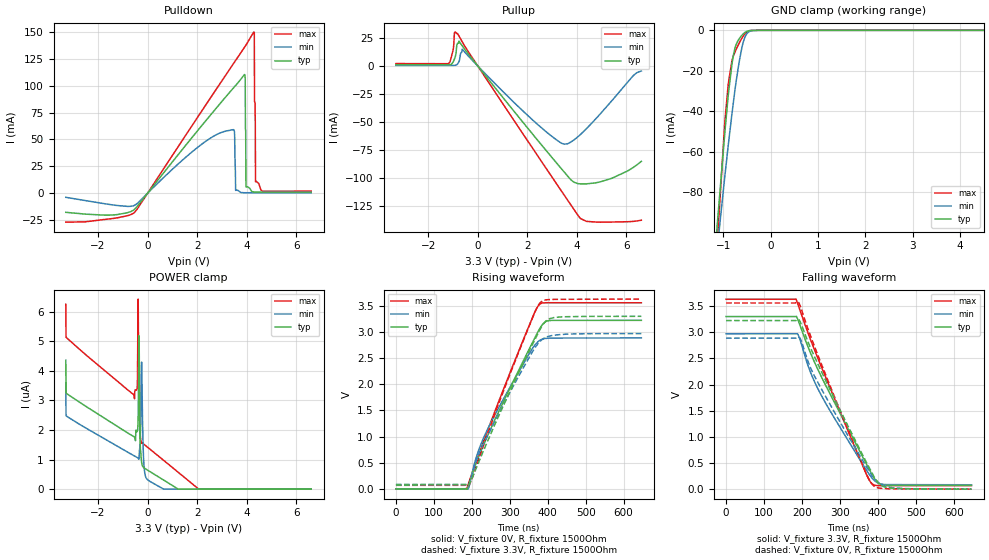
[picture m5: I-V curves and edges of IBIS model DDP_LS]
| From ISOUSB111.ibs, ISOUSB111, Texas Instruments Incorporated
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[Model]   DDP_LS
Model_type   I/O
Polarity   Non-Inverting
Enable   Active-Low
Vinl = 0.8
Vinh = 2
Vmeas = 1.65
Vref = 1.65
Cref = 7pF
Rref = 15000
|   typ   min   max
C_comp   8pF   5pF   10pF
[Voltage Range]   3.3   2.97   3.63
[Temperature Range]   27   150   -40
[Pullup Reference]   3.3   2.97   3.63
[Pulldown Reference]   -0   -0   -0
[Power Clamp Reference]   3.3   2.97   3.63
[GND Clamp Reference]   0   0   0
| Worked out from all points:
|   slope of the pulldown table from 0 to 0.495 V, typ, clamps not added: 34.2 ohm
|   slope of the pullup table from 0 to 0.495 V, typ, clamps not added: 35.8 ohm
|   GND clamp passes 1 mA (typ) near -0.54 V on its own axis
|   falling waveform, V_fixture 3.3V, R_fixture 1500Ohm: 20-80 % time 133ns typ, 130ns min, 121ns max; typ from 3.3 V to 0.073 V
|   rising waveform, V_fixture 0V, R_fixture 1500Ohm: 20-80 % time 125ns typ, 119ns min, 114ns max; typ from 0 V to 3.22 V
|   rising waveform, V_fixture 3.3V, R_fixture 1500Ohm: 20-80 % time 122ns typ, 124ns min, 112ns max; typ from 0.073 V to 3.3 V
|   falling waveform, V_fixture 0V, R_fixture 1500Ohm: 20-80 % time 130ns typ, 134ns min, 119ns max; typ from 3.22 V to 0 V
[Pulldown]
|   Voltage   I(typ)   I(min)   I(max)
-3.3V     -17.81mA   -3.846mA   -26.98mA
-537.9mV  -15.2mA    -11.4mA    -18.05mA
3.462V    97.83mA    59.07mA    120.4mA
3.551V    100.2mA    2.556mA    123.5mA
3.907V    110.2mA    416.6uA    135.6mA
3.937V    106.6mA    416.6uA    136.7mA
3.967V    5.838mA    416.6uA    137.7mA
4.283V    1.076mA    416.7uA    149.8mA
4.303V    991uA      416.7uA    149mA
4.313V    991.3uA    416.7uA    85.24mA
4.353V    991.6uA    416.7uA    10.59mA
6.6V      1.045mA    452.9uA    1.865mA
[GND Clamp]
|   Voltage   I(typ)   I(min)   I(max)
-3.3V     -1.286A    -1.121A    -1.579A
-1.3V     -145.3mA   -147.2mA   -170.6mA
-973.5mV  -52.59mA   -73.66mA   -47.68mA
-894.3mV  -32.06mA   -56.81mA   -26.49mA
-815.1mV  -16.5mA    -41.06mA   -14.88mA
-785.4mV  -12.23mA   -35.46mA   -12.65mA
-735.9mV  -7.575mA   -26.62mA   -9.853mA
-627mV    -3.033mA   -10.97mA   -4.745mA
-567.6mV  -1.539mA   -5.066mA   -2.489mA
-498.3mV  -471.8uA   -1.571mA   -746.6uA
-260.7mV  0A         -5.306uA   0A
6.6V      0A         0A         0A
[Pullup]
|   Voltage   I(typ)   I(min)   I(max)
-3.3V     1.143mA    463.3uA    2.099mA
-1.181V   1.062mA    442.6uA    2.004mA
-993.3mV  3.511mA    442.3uA    14.23mA
-933.9mV  6.5mA      535.6uA    29.94mA
-815.1mV  20.27mA    1.644mA    29.11mA
-627mV    18.08mA    14.98mA    21.69mA
1.957V    -54.05mA   -43.09mA   -65.15mA
3.491V    -95.05mA   -70.02mA   -115.7mA
3.868V    -103.9mA   -66.45mA   -128mA
4.382V    -105.5mA   -56.24mA   -139.1mA
5.412V    -100.5mA   -31.08mA   -139.7mA
6.6V      -85.4mA    -4.484mA   -138.1mA
[POWER Clamp]
|   Voltage   I(typ)   I(min)   I(max)
-3.3V     4.356uA    3.599uA    6.246uA
-3.29V    3.241uA    2.478uA    5.13uA
-528mV    1.757uA    1.119uA    3.051uA
-419.1mV  1.947uA    1.069uA    3.413uA
-379.5mV  2.484uA    1.044uA    6.42uA
-349.8mV  5.181uA    1.013uA    3.193uA
-310.2mV  1.898uA    1.42uA     1.946uA
-250.8mV  974.2nA    4.159uA    1.566uA
-171.6mV  741.4nA    1.215uA    1.531uA
-62.7mV   674.2nA    384.4nA    1.457uA
2.056V    0A         0A         4.445nA
6.6V      0A         0A         0A
[Ramp]
R_load = 1500
|   typ   min   max
dV/dt_r   1.93354/1.24911e-07   1.73136/1.18394e-07   2.13504/1.14552e-07
dV/dt_f   1.93557/1.33079e-07   1.73127/1.2979e-07   2.13707/1.21131e-07
[Falling Waveform]
V_fixture = 3.3V
V_fixture_min = 2.97V
V_fixture_max = 3.63V
R_fixture = 1500Ohm
C_fixture = 0F
|   Time   V(typ)   V(min)   V(max)
0s        3.299V     2.969V     3.629V
184.2ns   3.299V     2.971V     3.633V
191ns     3.206V     2.932V     3.498V
221.9ns   2.613V     2.245V     2.87V
251ns     2.15V      1.793V     2.34V
367.2ns   517.4mV    394.5mV    326.4mV
386.1ns   259.2mV    198.6mV    94.88mV
400.5ns   119.6mV    118mV      68.01mV
417.8ns   75.59mV    89.79mV    67.55mV
646.7ns   73.35mV    83.91mV    67.4mV
[Rising Waveform]
V_fixture = 0V
V_fixture_min = 0V
V_fixture_max = 0V
R_fixture = 1500Ohm
C_fixture = 0F
|   Time   V(typ)   V(min)   V(max)
0s        -34.15uV   -42.85uV   -28.52uV
186ns     -168.8uV   1.964mV    -4.172mV
191.3ns   67.7mV     9.248mV    102.6mV
214.5ns   547.9mV    666.1mV    585mV
246.8ns   1.101V     1.219V     1.216V
364.1ns   2.86V      2.73V      3.351V
380.6ns   3.085V     2.846V     3.54V
393.7ns   3.194V     2.876V     3.558V
410.5ns   3.222V     2.884V     3.559V
646.7ns   3.223V     2.886V     3.558V
[Rising Waveform]
V_fixture = 3.3V
V_fixture_min = 2.97V
V_fixture_max = 3.63V
R_fixture = 1500Ohm
C_fixture = 0F
|   Time   V(typ)   V(min)   V(max)
0s        73.35mV    83.91mV    67.4mV
192.6ns   79.15mV    74.4mV     72.28mV
216.9ns   488.5mV    643.3mV    541.5mV
251ns     1.07V      1.158V     1.241V
359.2ns   2.753V     2.614V     3.257V
376.2ns   3V         2.793V     3.522V
386.1ns   3.126V     2.859V     3.594V
400.5ns   3.238V     2.912V     3.618V
417.8ns   3.278V     2.939V     3.623V
646.7ns   3.299V     2.969V     3.629V
[Falling Waveform]
|Gnd
V_fixture = 0V
V_fixture_min = 0V
V_fixture_max = 0V
R_fixture = 1500Ohm
C_fixture = 0F
|   Time   V(typ)   V(min)   V(max)
0s        3.223V     2.886V     3.558V
191.3ns   3.239V     2.902V     3.567V
199.1ns   3.137V     2.819V     3.425V
222.8ns   2.697V     2.316V     2.926V
246.8ns   2.316V     1.974V     2.47V
371.6ns   488.3mV    407.7mV    264.4mV
391.1ns   226mV      201.1mV    52.04mV
404.8ns   95.88mV    109.6mV    19.13mV
427.6ns   25.02mV    42.81mV    7.952mV
646.7ns   -34.15uV   -42.85uV   -28.52uV
